|   IBIS Model of PowerPro PowerPC to SDRAM Memory Controller
[IBIS Ver]   3.2
[Comment char]  |_char
[File name]   a5000m21.ibs
[File Rev]   2.1
[Date]   June 2, 2002
[Source]   SPICE-to-IBIS translation
[Notes]
| Temperature: 25C typ, -40C max, 80C min.
|   Revision History:
   01 6/6/01 -- Initial release
   02 6/26/02 -- RLC and model_name updated.
   35A5000_MI002_02 release, Sept 2009 - updated for IDT formatting
[Disclaimer] This model is subject to change.
   Integrated Device Technology, Inc. ("IDT") hereby grants the
   user of this IBIS model a non-exclusive, nontransferable
   license to use this IBIS model under the following terms. The
   user is granted this license only to use the IBIS model and is
   not granted rights to sell, copy (except as needed to run the
   IBIS model), rent, lease or sub-license the IBIS model in
   whole or in part, or in modified form to anyone. The User may
   modify the IBIS model to suit its specific applications, but
   rights to derivative works and such modifications shall belong
   to IDT. This IBIS model is provided on an AS IS" basis and IDT
   makes absolutely no warranty with respect to the information
   contained herein. IDT DISCLAIMS AND CUSTOMER WAIVES ALL
   WARRANTIES, EXPRESS AND IMPLIED, INCLUDING WARRANTIES OF
   MERCHANTABILITY AND FITNESS FOR A PARTICULAR PURPOSE. THE
   ENTIRE RISK AS TO QUALITY AND PERFORMANCE IS WITH THE USER
   ACCORDINGLY, IN NO EVENT SHALL IDT BE LIABLE FOR ANY DIRECT OR
   INDIRECT DAMAGES, WHETHER IN CONTRACT OR TORT, INCLUDING ANY
   LOST PROFITS OR OTHER INCIDENTAL, CONSEQUENTIAL, EXEMPLARY, OR
   PUNITIVE DAMAGES ARISING OUT OF THE USE OR APPLICATION OF THE
   IBIS model. Further, IDT reserves the right to make changes
   without notice to any product herein to improve reliability,
   function, or design. IDT does not convey any license under
   patent rights or any other intellectual property rights,
   including those of third parties. IDT is not obligated to
   provide maintenance or support for the licensed IBIS model.
[Copyright]   Copyright 2009, Integrated Device Technology, Inc. all
   rights reserved.
|   COMPONENT: CA91L750
[Component]   CA91L750
[Manufacturer]  Integrated Device Technology, Inc.
[Package]
|   variable   typ   min   max
   R_pkg   81.9775m   22.0000m   163.0000m
   L_pkg   2.6613n   0.7800n   5.2100n
   C_pkg   1.1287p   0.8720p   1.6790p
|Package parameters for Lead including bondwire inductance
[Pin]   signal_name   model_name   R_pin   L_pin   C_pin
K4   BIDIR_CTRL   Input_model   32m   1.07n   1.087p
C16   EE_AL1   IO_buffer   80m   2.6n   1.31p
C15   EE_AL2   IO_buffer   54m   1.78n   0.996p
B15   EE_CS[0]   IO_buffer   80m   2.58n   1.046p
A15   EE_CS[1]   IO_buffer   94m   3.04n   0.986p
C14   EE_CS[2]   IO_buffer   48m   1.6n   0.932p
B14   EE_CS[3]   IO_buffer   73m   2.39n   0.988p
D12   EE_DATA[0]   IO_buffer   45m   1.49n   1.183p
A14   EE_DATA[1]   IO_buffer   90m   2.92n   0.952p
C13   EE_DATA[2]   IO_buffer   43m   1.44n   0.917p
B13   EE_DATA[3]   IO_buffer   69m   2.24n   0.95p
A13   EE_DATA[4]   IO_buffer   85m   2.77n   0.911p
C12   EE_DATA[5]   IO_buffer   43m   1.43n   0.886p
B12   EE_DATA[6]   IO_buffer   68m   2.21n   0.955p
A12   EE_DATA[7]   IO_buffer   85m   2.76n   0.909p
A17   EE_OE_b   IO_buffer   110m   3.54n   1.129p
A16   EE_READY   IO_buffer   105m   3.39n   1.081p
D14   EE_RNW   IO_buffer   42m   1.41n   1.175p
B16   EE_WE_b   IO_buffer   83m   2.68n   1.073p
A5   EXT_INT_b   IO_buffer   102m   3.29n   1.053p
D7   HRESET_b   IO_buffer   59m   1.94n   1.332p
B10   I2C0_SCLK   IO_buffer   62m   2.04n   0.937p
C10   I2C0_SDA   IO_buffer   42m   1.42n   0.985p
A9   I2C1_SCLK   IO_buffer   87m   2.82n   0.924p
B9   I2C1_SDA   IO_buffer   64m   2.08n   0.922p
Y20   JT_TCK   Input_model   89m   2.89n   1.352p
W5   JT_TDI   Input_model   68m   2.21n   1.38p
W22   JT_TDO   IO_buffer   121m   3.9n   1.221p
D1   JT_TMS   Input_model   123m   3.95n   1.235p
A8   JT_TRST_b   Input_model   88m   2.84n   0.928p
W8   PB_A[0]   IO_buffer   31m   1.06n   0.967p
AA5   PB_A[1]   IO_buffer   112m   3.61n   1.326p
AB7   PB_A[10]   IO_buffer   116m   3.74n   1.178p
AA8   PB_A[11]   IO_buffer   90m   2.9n   1.131p
AB8   PB_A[12]   IO_buffer   105m   3.39n   1.08p
Y9   PB_A[13]   IO_buffer   58m   1.9n   1.02p
AA9   PB_A[14]   IO_buffer   84m   2.72n   1.066p
AB9   PB_A[15]   IO_buffer   96m   3.11n   1.022p
Y10   PB_A[16]   IO_buffer   53m   1.76n   0.88p
AA10   PB_A[17]   IO_buffer   76m   2.47n   1.028p
AB10   PB_A[18]   IO_buffer   93m   3.01n   0.984p
AB11   PB_A[19]   IO_buffer   92m   2.99n   0.978p
Y6   PB_A[2]   IO_buffer   84m   2.72n   1.277p
Y11   PB_A[20]   IO_buffer   49m   1.64n   0.94p
AA11   PB_A[21]   IO_buffer   73m   2.37n   0.983p
AB12   PB_A[22]   IO_buffer   84m   2.73n   0.897p
AA12   PB_A[23]   IO_buffer   62m   2.05n   0.899p
Y12   PB_A[24]   Input_model   47m   1.55n   1.003p
AB13   PB_A[25]   Input_model   87m   2.82n   0.923p
AA13   PB_A[26]   Input_model   67m   2.19n   0.946p
Y13   PB_A[27]   Input_model   49m   1.63n   0.949p
AB14   PB_A[28]   Input_model   95m   3.06n   0.989p
AA14   PB_A[29]   Input_model   76m   2.47n   1.002p
AB5   PB_A[3]   IO_buffer   125m   4.02n   1.252p
AB15   PB_A[30]   Input_model   93m   3.02n   0.978p
Y14   PB_A[31]   Input_model   50m   1.65n   0.983p
AA6   PB_A[4]   IO_buffer   100m   3.24n   1.225p
Y7   PB_A[5]   IO_buffer   74m   2.42n   1.204p
AB6   PB_A[6]   IO_buffer   115m   3.72n   1.17p
AA7   PB_A[7]   IO_buffer   89m   2.89n   1.145p
W9   PB_A[8]   IO_buffer   39m   1.29n   1.152p
Y8   PB_A[9]   IO_buffer   62m   2.03n   1.196p
C5   PB_AACK_b   IO_buffer   63m   2.06n   1.059p
AA15   PB_AP[0]   IO_buffer   73m   2.39n   1.001p
W14   PB_AP[1]   IO_buffer   30m   1.02n   1.045p
AB16   PB_AP[2]   IO_buffer   98m   3.15n   1.016p
Y15   PB_AP[3]   IO_buffer   54m   1.79n   1.086p
B4   PB_ARTRY_b   IO_buffer   131m   4.2n   1.301p
AB3   PB_BG[0]   IO_buffer   138m   4.41n   1.364p
AA4   PB_BG[1]   IO_buffer   111m   3.56n   1.336p
W7   PB_BR[0]   IO_buffer   23m   0.79n   0.983p
Y4   PB_BR[1]   IO_buffer   94m   3.04n   1.356p
A3   PB_CLK   Clock_buffer   113m   3.65n   1.149p
C6   PB_D[0]   IO_buffer   55m   1.8n   1.092p
B5   PB_D[1]   IO_buffer   84m   2.74n   1.1p
C2   PB_D[10]   IO_buffer   137m   4.4n   1.531p
E4   PB_D[11]   IO_buffer   41m   1.38n   1.342p
D3   PB_D[12]   IO_buffer   81m   2.63n   1.197p
C1   PB_D[13]   IO_buffer   136m   4.36n   1.345p
D2   PB_D[14]   IO_buffer   149m   4.78n   1.461p
F4   PB_D[15]   IO_buffer   45m   1.49n   1.086p
E3   PB_D[16]   IO_buffer   74m   2.42n   1.164p
H4   PB_D[17]   IO_buffer   40m   1.34n   1.265p
E2   PB_D[18]   IO_buffer   95m   3.08n   1.202p
F3   PB_D[19]   IO_buffer   67m   2.18n   1.167p
A4   PB_D[2]   IO_buffer   112m   3.6n   1.138p
E1   PB_D[20]   IO_buffer   112m   3.6n   1.139p
F2   PB_D[21]   IO_buffer   84m   2.74n   1.113p
G3   PB_D[22]   IO_buffer   59m   1.94n   1.046p
F1   PB_D[23]   IO_buffer   105m   3.38n   1.076p
G2   PB_D[24]   IO_buffer   78m   2.54n   1.049p
J4   PB_D[25]   IO_buffer   40m   1.34n   1.153p
H3   PB_D[26]   IO_buffer   56m   1.84n   1.017p
G1   PB_D[27]   IO_buffer   103m   3.34n   1.066p
H2   PB_D[28]   IO_buffer   76m   2.48n   1.067p
J3   PB_D[29]   IO_buffer   54m   1.78n   1.087p
D6   PB_D[3]   IO_buffer   37m   1.25n   1.164p
H1   PB_D[30]   IO_buffer   101m   3.26n   1.044p
J2   PB_D[31]   IO_buffer   73m   2.39n   1.004p
J1   PB_D[32]   IO_buffer   94m   3.04n   0.986p
K3   PB_D[33]   IO_buffer   52m   1.7n   0.964p
K2   PB_D[34]   IO_buffer   70m   2.27n   0.985p
K1   PB_D[35]   IO_buffer   91m   2.96n   0.961p
L1   PB_D[36]   IO_buffer   88m   2.84n   0.93p
L2   PB_D[37]   IO_buffer   70m   2.28n   0.943p
L3   PB_D[38]   IO_buffer   50m   1.65n   0.948p
M1   PB_D[39]   IO_buffer   84m   2.71n   0.895p
A1   PB_D[4]   IO_buffer   163m   5.21n   1.679p
M2   PB_D[40]   IO_buffer   63m   2.05n   0.897p
M3   PB_D[41]   IO_buffer   46m   1.54n   0.944p
N1   PB_D[42]   IO_buffer   84m   2.73n   0.901p
N2   PB_D[43]   IO_buffer   65m   2.13n   0.916p
N3   PB_D[44]   IO_buffer   52m   1.72n   0.965p
P1   PB_D[45]   IO_buffer   90m   2.91n   0.949p
P2   PB_D[46]   IO_buffer   71m   2.31n   0.958p
R1   PB_D[47]   IO_buffer   94m   3.05n   1p
P3   PB_D[48]   IO_buffer   54m   1.77n   1.029p
P4   PB_D[49]   IO_buffer   42m   1.41n   1.125p
B2   PB_D[5]   IO_buffer   125m   4.03n   1.536p
T1   PB_D[50]   IO_buffer   96m   3.11n   1.023p
R3   PB_D[51]   IO_buffer   53m   1.74n   1.035p
T2   PB_D[52]   IO_buffer   77m   2.5n   1.021p
U1   PB_D[53]   IO_buffer   101m   3.25n   1.04p
T3   PB_D[54]   IO_buffer   58m   1.92n   1.054p
U2   PB_D[55]   IO_buffer   85m   2.75n   1.076p
V1   PB_D[56]   IO_buffer   108m   3.48n   1.104p
R4   PB_D[57]   IO_buffer   45m   1.49n   1.188p
U3   PB_D[58]   IO_buffer   64m   2.09n   1.098p
V2   PB_D[59]   IO_buffer   91m   2.93n   1.158p
C3   PB_D[6]   IO_buffer   86m   2.78n   1.613p
W1   PB_D[60]   IO_buffer   117m   3.77n   1.186p
Y1   PB_D[61]   IO_buffer   126m   4.06n   1.262p
U4   PB_D[62]   IO_buffer   48m   1.6n   1.124p
V3   PB_D[63]   IO_buffer   72m   2.35n   1.159p
D4   PB_D[7]   IO_buffer   47m   1.55n   1.309p
B1   PB_D[8]   IO_buffer   137m   4.38n   1.354p
G4   PB_D[9]   IO_buffer   50m   1.66n   1.343p
Y5   PB_DBG[0]   IO_buffer   84m   2.74n   1.319p
W6   PB_DBG[1]   IO_buffer   64m   2.11n   1.344p
T4   PB_DP[0]   IO_buffer   44m   1.48n   1.202p
W2   PB_DP[1]   IO_buffer   98m   3.15n   1.273p
V4   PB_DP[2]   IO_buffer   54m   1.78n   1.187p
W3   PB_DP[3]   IO_buffer   83m   2.68n   1.254p
Y2   PB_DP[4]   IO_buffer   110m   3.56n   1.312p
AA1   PB_DP[5]   IO_buffer   131m   4.2n   1.326p
AB1   PB_DP[6]   IO_buffer   143m   4.58n   1.408p
AA2   PB_DP[7]   IO_buffer   117m   3.78n   1.371p
Y3   PB_DVAL_b   IO_buffer   90m   2.92n   1.313p
AA3   PB_INT_b   IO_buffer   111m   3.59n   1.33p
W4   PB_TA_b   IO_buffer   75m   2.43n   1.436p
B7   PB_TBST_b   Input_model   71m   2.31n   0.96p
AB2   PB_TEA_b   IO_buffer   137m   4.39n   1.356p
AB4   PB_TS_b   Input_model   131m   4.2n   1.309p
A6   PB_TSIZ[0]   Input_model   111m   3.58n   1.134p
C7   PB_TSIZ[1]   Input_model   128m   4.1n   1.302p
B6   PB_TSIZ[2]   Input_model   76m   2.46n   1.057p
D8   PB_TSIZ[3]   Input_model   44m   1.47n   1.189p
C9   PB_TT[0]   Input_model   47m   1.56n   1.045p
B8   PB_TT[1]   Input_model   67m   2.18n   0.936p
D9   PB_TT[2]   Input_model   42m   1.39n   1.176p
A7   PB_TT[3]   Input_model   90m   2.92n   1.126p
C8   PB_TT[4]   Input_model   50m   1.65n   1.059p
AA16   PO_RANGE   Input_model   81m   2.62n   1.053p
N19   PORESET_b   Input_model   26m   0.9n   0.966p
W15   SD_A[0]   IO_buffer   44m   1.45n   1.163p
AB19   SD_A[1]   IO_buffer   126m   4.04n   1.281p
Y19   SD_A[10]   IO_buffer   78m   2.54n   1.23p
AA20   SD_A[11]   IO_buffer   103m   3.33n   1.291p
AB21   SD_A[12]   IO_buffer   131m   4.2n   1.326p
Y17   SD_A[2]   IO_buffer   70m   2.29n   1.33p
AA18   SD_A[3]   IO_buffer   96m   3.12n   1.189p
W17   SD_A[4]   IO_buffer   63m   2.06n   1.212p
W16   SD_A[5]   IO_buffer   34m   1.15n   1.027p
Y18   SD_A[6]   IO_buffer   75m   2.45n   1.191p
AA19   SD_A[7]   IO_buffer   102m   3.29n   1.272p
AB20   SD_A[8]   IO_buffer   128m   4.1n   1.298p
W18   SD_A[9]   IO_buffer   53m   1.74n   1.292p
AB22   SD_BA[0]   IO_buffer   142m   4.56n   1.425p
AA21   SD_BA[1]   IO_buffer   116m   3.74n   1.383p
AB18   SD_CAS_b   IO_buffer   118m   3.78n   1.189p
V20   SD_CS[0]   IO_buffer   76m   2.47n   1.186p
U19   SD_CS[1]   IO_buffer   56m   1.83n   1.154p
R19   SD_CS[2]   IO_buffer   28m   0.98n   0.959p
V21   SD_CS[3]   IO_buffer   106m   3.41n   1.272p
U20   SD_CS[4]   IO_buffer   70m   2.28n   1.142p
V22   SD_CS[5]   IO_buffer   120m   3.86n   1.209p
U21   SD_CS[6]   IO_buffer   94m   3.05n   1.17p
T20   SD_CS[7]   IO_buffer   60m   1.97n   1.044p
U22   SD_D[0]   IO_buffer   107m   3.44n   1.095p
T21   SD_D[1]   IO_buffer   82m   2.67n   1.068p
N20   SD_D[10]   IO_buffer   54m   1.78n   1.048p
N21   SD_D[11]   IO_buffer   75m   2.44n   1.009p
N22   SD_D[12]   IO_buffer   91m   2.95n   0.962p
M21   SD_D[13]   IO_buffer   65m   2.14n   0.92p
M20   SD_D[14]   IO_buffer   50m   1.67n   0.913p
M22   SD_D[15]   IO_buffer   84m   2.72n   0.895p
L22   SD_D[16]   IO_buffer   81m   2.63n   0.872p
L21   SD_D[17]   IO_buffer   61m   1.99n   0.887p
L20   SD_D[18]   IO_buffer   46m   1.53n   0.898p
K22   SD_D[19]   IO_buffer   84m   2.72n   0.896p
P19   SD_D[2]   IO_buffer   27m   0.94n   0.939p
K21   SD_D[20]   IO_buffer   66m   2.14n   0.926p
K20   SD_D[21]   IO_buffer   48m   1.58n   0.949p
J22   SD_D[22]   IO_buffer   90m   2.92n   0.951p
J21   SD_D[23]   IO_buffer   73m   2.39n   0.991p
H22   SD_D[24]   IO_buffer   89m   2.9n   0.944p
J20   SD_D[25]   IO_buffer   46m   1.53n   0.932p
H21   SD_D[26]   IO_buffer   74m   2.41n   0.988p
J19   SD_D[27]   IO_buffer   27m   0.93n   1.019p
G22   SD_D[28]   IO_buffer   99m   3.21n   1.029p
H20   SD_D[29]   IO_buffer   50m   1.64n   0.966p
R20   SD_D[3]   IO_buffer   59m   1.93n   1.035p
G21   SD_D[30]   IO_buffer   74m   2.42n   1.012p
F22   SD_D[31]   IO_buffer   102m   3.3n   1.054p
F21   SD_D[32]   IO_buffer   86m   2.78n   1.097p
H19   SD_D[33]   IO_buffer   44m   1.45n   1.165p
E22   SD_D[34]   IO_buffer   105m   3.38n   1.077p
F20   SD_D[35]   IO_buffer   63m   2.05n   1.096p
E21   SD_D[36]   IO_buffer   91m   2.93n   1.149p
D22   SD_D[37]   IO_buffer   113m   3.65n   1.149p
F19   SD_D[38]   IO_buffer   50m   1.65n   1.109p
E20   SD_D[39]   IO_buffer   72m   2.34n   1.171p
T22   SD_D[4]   IO_buffer   110m   3.54n   1.122p
D21   SD_D[40]   IO_buffer   99m   3.21n   1.227p
G19   SD_D[41]   IO_buffer   44m   1.46n   1.177p
C22   SD_D[42]   IO_buffer   122m   3.93n   1.251p
E19   SD_D[43]   IO_buffer   52m   1.7n   1.135p
D20   SD_D[44]   IO_buffer   78m   2.52n   1.22p
C21   SD_D[45]   IO_buffer   101m   3.26n   1.261p
B22   SD_D[46]   IO_buffer   128m   4.12n   1.303p
A22   SD_D[47]   IO_buffer   143m   4.58n   1.429p
B21   SD_D[48]   IO_buffer   118m   3.78n   1.397p
C20   SD_D[49]   IO_buffer   89m   2.9n   1.319p
R21   SD_D[5]   IO_buffer   85m   2.77n   1.108p
D19   SD_D[50]   IO_buffer   82m   2.66n   1.528p
A21   SD_D[51]   IO_buffer   137m   4.39n   1.378p
B20   SD_D[52]   IO_buffer   109m   3.53n   1.332p
D16   SD_D[53]   IO_buffer   22m   0.78n   0.976p
C19   SD_D[54]   IO_buffer   94m   3.05n   1.348p
D18   SD_D[55]   IO_buffer   55m   1.81n   1.167p
A20   SD_D[56]   IO_buffer   140m   4.5n   1.407p
B19   SD_D[57]   IO_buffer   112m   3.62n   1.343p
C18   SD_D[58]   IO_buffer   83m   2.69n   1.261p
A19   SD_D[59]   IO_buffer   127m   4.07n   1.267p
P20   SD_D[6]   IO_buffer   60m   1.98n   1.138p
D15   SD_D[60]   IO_buffer   29m   0.99n   0.945p
B18   SD_D[61]   IO_buffer   108m   3.48n   1.304p
C17   SD_D[62]   IO_buffer   84m   2.71n   1.289p
A18   SD_D[63]   IO_buffer   122m   3.94n   1.235p
R22   SD_D[7]   IO_buffer   109m   3.5n   1.111p
P21   SD_D[8]   IO_buffer   83m   2.69n   1.08p
P22   SD_D[9]   IO_buffer   99m   3.19n   1.026p
W19   SD_ECC[0]   IO_buffer   102m   3.29n   1.536p
AA22   SD_ECC[1]   IO_buffer   138m   4.44n   1.365p
Y21   SD_ECC[2]   IO_buffer   109m   3.5n   1.296p
W20   SD_ECC[3]   IO_buffer   77m   2.49n   1.199p
T19   SD_ECC[4]   IO_buffer   44m   1.48n   1.175p
V19   SD_ECC[5]   IO_buffer   86m   2.77n   1.522p
Y22   SD_ECC[6]   IO_buffer   135m   4.32n   1.337p
W21   SD_ECC[7]   IO_buffer   107m   3.45n   1.292p
AB17   SD_RAS_b   IO_buffer   108m   3.49n   1.11p
B17   SD_SELECT   IO_buffer   94m   3.05n   1.186p
AA17   SD_WE_b   IO_buffer   91m   2.94n   1.127p
C11   UART0_RX   IO_buffer   43m   1.44n   0.979p
A11   UART0_TX   IO_buffer   87m   2.83n   0.928p
A10   UART1_RX   IO_buffer   89m   2.87n   0.939p
B11   UART1_TX   IO_buffer   68m   2.22n   0.981p
| Models and submodels in the file (3): IO_buffer (I/O), Clock_buffer (Input), Input_model (Input)
